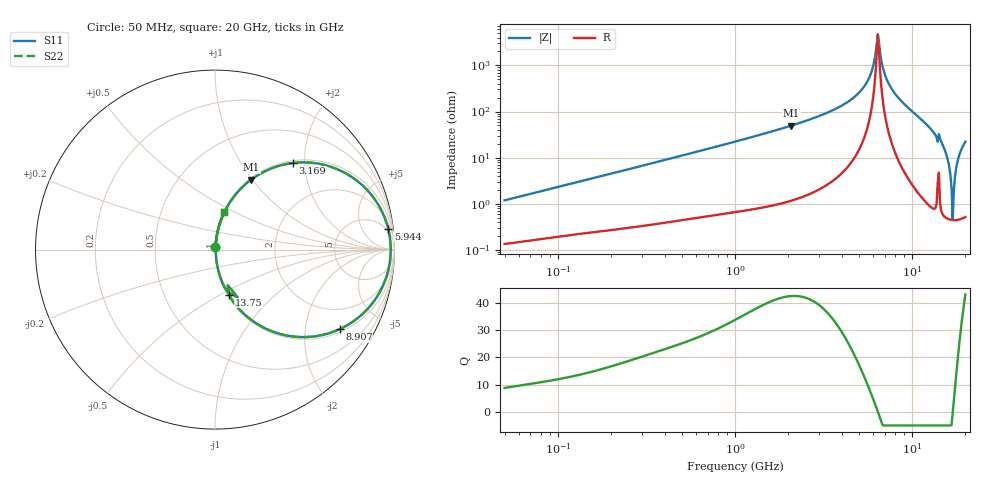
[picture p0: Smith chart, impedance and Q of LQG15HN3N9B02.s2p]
!Murata Part Number: LQG15HN3N9B02
!These Parameters are Measured in Series Mode Connection
!  o--[Z]--o
!Port1  Port2
!  o-------o
!Freq. Start=50[MHz] Stop=20[GHz], 401[Steps]
# Hz S RI R 50
!Freq.(Hz) S11(Real) S11(Imag) S21(Real) S21(Imag) S12(Real) S12(Imag) S22(Real) S22(Imag)
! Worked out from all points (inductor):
!   401 points, 50 MHz to 20 GHz, reference 50 ohm
!   read as one part in series: L = 3.72 nH near 51.52 MHz
!   highest Q = 42.4 at 2.083 GHz (marker M1), where L = 3.79 nH
!   self-resonance near 6.407 GHz
!   S11 on the Smith chart (normalised r, x): 50 MHz: 1.00, +0.02; 3.169 GHz: 1.05, +1.75; 5.944 GHz: 4, +16; 8.907 GHz: 1.11, -3.05; 13.75 GHz: 1.02, -0.55; 20 GHz: 1.01, +0.44
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5e7  0.00149 0.0118  0.9985 -0.0118  0.9985 -0.0118  0.00149 0.0118
1.364002e8  0.0032 0.0308  0.9968 -0.0308  0.9968 -0.0308  0.0032 0.0308
3.721004e8  0.0104 0.0814  0.9896 -0.0814  0.9896 -0.0814  0.0104 0.0814
1e9  0.0526 0.2088  0.9474 -0.2088  0.9474 -0.2088  0.0526 0.2088
2.083303e9  0.2028 0.3905  0.7972 -0.3905  0.7972 -0.3905  0.2028 0.3905
2.728004e9  0.3333 0.4593  0.6667 -0.4593  0.6667 -0.4593  0.3333 0.4593
3.168813e9  0.4351 0.4827  0.5649 -0.4827  0.5649 -0.4827  0.4351 0.4827
4.81993e9  0.8176 0.3616  0.1824 -0.3616  0.1824 -0.3616  0.8176 0.3616
5.515528e9  0.9264 0.2198  0.0736 -0.2198  0.0736 -0.2198  0.9264 0.2198
5.944466e9  0.9647 0.1168  0.0353 -0.1168  0.0353 -0.1168  0.9647 0.1168
6.406762e9  0.9791 0.00112  0.0209 -0.00112  0.0209 -0.00112  0.9791 0.00112
7.009217e9  0.9574 -0.1441  0.0426 0.1441  0.0426 0.1441  0.9574 -0.1441
7.442007e9  0.9177 -0.2372  0.0823 0.2372  0.0823 0.2372  0.9177 -0.2372
8.907419e9  0.6938 -0.4437  0.3062 0.4437  0.3062 0.4437  0.6938 -0.4437
1.098561e10  0.3528 -0.4671  0.6472 0.4671  0.6472 0.4671  0.3528 -0.4671
1.375312e10  0.078 -0.2504  0.922 0.2504  0.922 0.2504  0.078 -0.2504
1.550395e10  0.0206 -0.1235  0.9794 0.1235  0.9794 0.1235  0.0206 -0.1235
1.646126e10  0.00624 -0.0416  0.9938 0.0416  0.9938 0.0416  0.00624 -0.0416
1.696185e10  0.00441 -0.00104  0.9956 0.00104  0.9956 0.00104  0.00441 -0.00104
1.747767e10  0.00593 0.0391  0.9941 -0.0391  0.9941 -0.0391  0.00593 0.0391
1.828096e10  0.0142 0.098  0.9858 -0.098  0.9858 -0.098  0.0142 0.098
2e10  0.0512 0.2091  0.9488 -0.2091  0.9488 -0.2091  0.0512 0.2091
